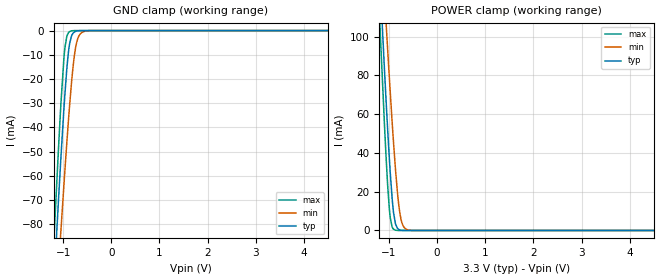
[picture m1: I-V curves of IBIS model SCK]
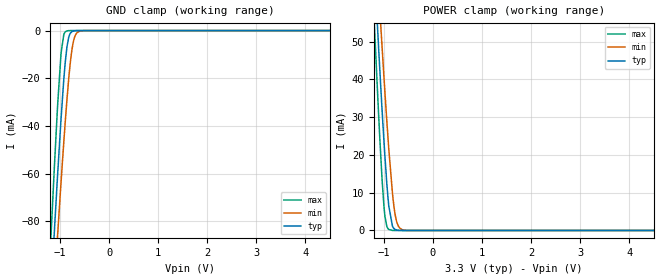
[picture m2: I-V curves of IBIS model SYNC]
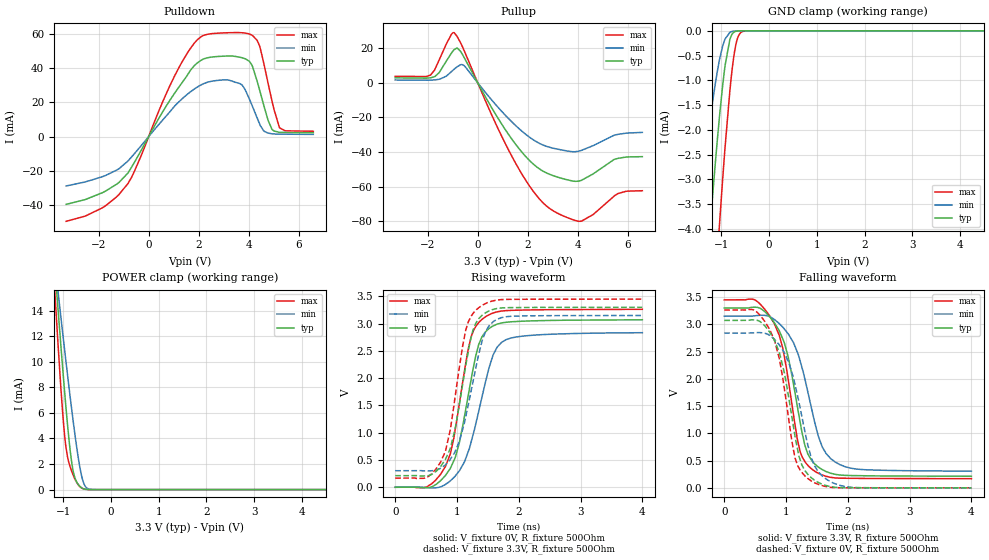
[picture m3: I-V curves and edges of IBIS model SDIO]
| Texas Instruments Incorporated
| Low-Noise Clock Jitter Cleaner with Dual Loop PLLs
| Marketing part#   Voltage Range   Package-type   #pins/pkg drawing
| LMK04826   3.0V - 3.6V   LLP   64-pin SQ
[IBIS Ver]   4.1
[File name]   lmk04826.ibs
[File Rev]   1.2
[Date]   04/24/2014
[Source]   Model built from spectre simulations at:
   Texas Instruments Incorporated.
   Analog-eLab, HPA
   12500 TI Blvd
   Dallas, TX -75243
   For Support e-mail: elab_ibis@list.ti.com
[Notes]   Revision History
   Rev 1.2: 04/24/2014
   - Correct LCPECL model name
   Rev 1.1: 01/28/2014
   - Add SYNC pin. Assign RESET to SDIO buffer
   Rev 1.0: 06/19/2013
   -Pulldown non-monotonic for LVDS_OSC model
   -Pulldown & pullup non-monotonic for LVPECL_OSC models
   -Pulldown & pullup non-monotonic for SDIO models
   -LVPECL simulation recommendation:
   It is recommended that a small (1nF or less) AC coupling cap
   be used. Larger values will result in long settling times
   - ccomp values are based on PVT settings:
   MIN: Low Voltage, High Temperature, Weak Process
   TYP: Nominal Voltage, Nominal Temperature, Nominal Process
   MAX: High Voltage, Low Temperature, Fast Process
   - C_comp although listed in numerical order of value are obtained from varying PVT conditions.
   For PVT conditions for each specific value, refer to the buffer description under respective [Model].
   IBIS model user is responsible for using appropriate C_comp to simulate for Signal Integrity.
[Disclaimer]  This model is designed as an aid for customers of Texas Instruments
 TI and its licensors and suppliers make no warranties, either expressed
 or implied, with respect to this  model, including the warranties of
 merchantability or fitness for a particular purpose.
 The model is provided solely on an "as is" basis. The entire risk as to
 its quality and performance is with the customer.
[Copyright] (C)Copyright 2014 Texas Instruments Incorporated.
   All rights reserved.
[Component]   LMK04826BISQ
[Manufacturer]  Texas Instruments Incorporated
[Package]   |64-pin LLP SQ package
|   typ   min   max
R_pkg   0   0   0
L_pkg   0   0   0
C_pkg   0   0   0
[Pin]   signal_name   model_name   R_pin   L_pin   C_pin
1   DCLKOUT0   TRI_MODE_OUT
2   DCLKOUT0*   TRI_MODE_OUT
3   SDCLKOUT1*   TRI_MODE_OUT
4   SDCLKOUT1   TRI_MODE_OUT
5   RESET   SDIO
6   SYNC   SYNC
7   NC   NC
8   NC   NC
9   NC   NC
10   VCC1   POWER
11   LDOBYP1   NC
12   LDOBYP2   NC
13   SDCLKOUT3   TRI_MODE_OUT
14   SDCLKOUT3*   TRI_MODE_OUT
15   DLKOUT2   TRI_MODE_OUT
16   DLKOUT2*   TRI_MODE_OUT
17   VCC2   POWER
18   CS   SCK
19   SCK   SCK
20   SDIO   SDIO
21   VCC3   POWER
22   SDCLKOUT5   TRI_MODE_OUT
23   SDCLKOUT5*   TRI_MODE_OUT
24   DLKOUT4   TRI_MODE_OUT
25   DLKOUT4*   TRI_MODE_OUT
26   VCC4   POWER
27   DLKOUT6   TRI_MODE_OUT
28   DLKOUT6*   TRI_MODE_OUT
29   SDCLKOUT7   TRI_MODE_OUT
30   SDCLKOUT7*   TRI_MODE_OUT
31   STATUS   SDIO
32   CPOUT1   NC
33   VCC5   POWER
34   CLKIN1   CLKIN
35   CLKIN1*   CLKIN
36   VCC6   POWER
37   CLKIN0   CLKIN
38   CLKIN0*   CLKIN
39   VCC7   POWER
40   OSCOUT   OSCOUT
41   OSCOUT*   OSCOUT
42   VCC8   POWER
43   OSCIN   OSCIN
44   OSCIN*   OSCIN
45   VCC9   POWER
46   CPOUT2   NC
47   VCC10   POWER
48   STATUS_LD2   SDIO
49   SDCLKOUT9   TRI_MODE_OUT
50   SDCLKOUT9*   TRI_MODE_OUT
51   DCLKOUT8   TRI_MODE_OUT
52   DCLKOUT8*   TRI_MODE_OUT
53   VCC11   POWER
54   DCLKOUT10   TRI_MODE_OUT
55   DCLKOUT10*   TRI_MODE_OUT
56   SDCLKOUT11   TRI_MODE_OUT
57   SDCLKOUT11*   TRI_MODE_OUT
58   CLKN_SEL0   NC
59   CLKN_SEL1   NC
60   SDCLKOUT13   TRI_MODE_OUT
61   SDCLKOUT13*   TRI_MODE_OUT
62   DCLKOUT12   TRI_MODE_OUT
63   DCLKOUT12*   TRI_MODE_OUT
64   VCC12   POWER
[Diff pin]  inv_pin  vdiff  tdelay_typ  tdelay_min  tdelay_max
 1   2   0.0   0.0s   0.0s   0.0s
 4   3   0.0   0.0s   0.0s   0.0s
13   14   0.0   0.0s   0.0s   0.0s
15   16   0.0   0.0s   0.0s   0.0s
22   23   0.0   0.0s   0.0s   0.0s
24   25   0.0   0.0s   0.0s   0.0s
27   28   0.0   0.0s   0.0s   0.0s
29   30   0.0   0.0s   0.0s   0.0s
34   35   0.0   0.0s   0.0s   0.0s
37   38   0.0   0.0s   0.0s   0.0s
40   41   0.0   0.0s   0.0s   0.0s
43   44   0.0   0.0s   0.0s   0.0s
49   50   0.0   0.0s   0.0s   0.0s
51   52   0.0   0.0s   0.0s   0.0s
54   55   0.0   0.0s   0.0s   0.0s
56   57   0.0   0.0s   0.0s   0.0s
60   61   0.0   0.0s   0.0s   0.0s
62   63   0.0   0.0s   0.0s   0.0s
[Model Selector] TRI_MODE_OUT
LVDS   LVDS OUTPUT
HSDS_6mA   HSDS 6mA OUTPUT
HSDS_8mA   HSDS 8mA OUTPUT
HSDS_10mA   HSDS 10mA OUTPUT
LVPECL1P6   LVPECL 1.6V OUTPUT
LVPECL2P0   LVPECL 2.0V OUTPUT
LCPECL   LCPECL
[Model Selector] OSCOUT
LVPECL1P6_OSC   LVPECL 1.6V OUTPUT
LVPECL2P0_OSC   LVPECL 2.0V OUTPUT
LVDS_OSC   LVDS OUTPUT
LVCMOS_OSC   LVCMOS OUTPUT
[Define Package Model]  llp64_lmk04826nsa2
[Manufacturer]  Unknown
[OEM]  Unknown
[Description]  Package Model,10GHz using buildsheet AD#LMK04826NSA2-01 RevA
[Number Of Pins]  65
[Pin Numbers]
|Pin Num   Terminal Name
1   | L1:1
2   | L2:2
3   | L3:3
4   | L4:4
5   | L5:5
6   | L6:6
7   | L7:7
8   | L8:8
9   | L9:9
10   | L10:10
11   | L11:11
12   | L12:12
13   | L13:13
14   | L14:14
15   | L15:15
16   | L16:16
17   | L17:17
18   | L18:18
19   | L19:19
20   | L20:20
21   | L21:21
22   | L22:22
23   | L23:23
24   | L24:24
25   | L25:25
26   | L26:26
27   | L27:27
28   | L28:28
29   | L29:29
30   | L30:30
31   | L31:31
32   | L32:32
33   | L33:33
34   | L34:34
35   | L35:35
36   | L36:36
37   | L37:37
38   | L38:38
39   | L39:39
40   | L40:40
41   | L41:41
42   | L42:42
43   | L43:43
44   | L44:44
45   | L45:45
46   | L46:46
47   | L47:47
48   | L48:48
49   | L49:49
50   | L50:50
51   | L51:51
52   | L52:52
53   | L53:53
54   | L54:54
55   | L55:55
56   | L56:56
57   | L57:57
58   | L58:58
59   | L59:59
60   | L60:60
61   | L61:61
62   | L62:62
63   | L63:63
64   | L64:64
65   | LDAP:65
[Model Data]
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[End Model Data]
[End Package Model]
| Models and submodels in the file (16): SCK (Input), SYNC (Input), SDIO (I/O), CLKIN (Input), OSCIN (Input), LVCMOS_OSC (Output), LVDS_OSC (Output), LVPECL1P6_OSC (Output), LVPECL2P0_OSC (Output), LVDS (Output), HSDS_6mA (Output), HSDS_8mA (Output), HSDS_10mA (Output), LVPECL1P6 (Output), LVPECL2P0 (Output), LCPECL (Output)
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|   Model SCK
[Model]   SCK
Model_type   Input
Vinl = 0.4
Vinh = 1.6
|   typ   min   max
|   (nom PVT)   (fast PVT)   (slow PVT)
C_comp   0.5966pF   0.57765pF   0.6104pF
[Voltage Range]   3.3   3.15   3.45
[Temperature Range]   27   125   -40
[Power Clamp Reference]   3.3   3.15   3.45
[GND Clamp Reference]   0   0   0
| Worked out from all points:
|   GND clamp passes 1 mA (typ) near -0.79 V on its own axis
|   POWER clamp passes 1 mA (typ) near -0.82 V on its own axis
[GND Clamp]
|   Voltage   I(typ)   I(min)   I(max)
-3.3V     -942.6mA   -854.7mA   -1.024A
-1.181V   -100.7mA   -125.5mA   -82.33mA
-1.092V   -68.4mA    -97.02mA   -46.97mA
-1.043V   -51.28mA   -81.58mA   -28.98mA
-963.6mV  -26.25mA   -57.73mA   -7.074mA
-924mV    -15.81mA   -46.4mA    -2.338mA
-864.6mV  -5.241mA   -30.59mA   -416.6uA
-785.4mV  -906.4uA   -13.39mA   -21.05uA
-726mV    -220.2uA   -5.463mA   -1.21uA
-656.7mV  -28.09uA   -1.707mA   0A
-537.9mV  -325.8nA   -217.8uA   0A
6.59V     0A         0A         0A
[POWER Clamp]
|   Voltage   I(typ)   I(min)   I(max)
-3.3V     1.303A     1.181A     1.417A
-1.191V   132mA      165.3mA    107.9mA
-1.181V   126.9mA    160.8mA    102.3mA
-1.092V   82.42mA    121.3mA    53.89mA
-1.063V   68.26mA    108.5mA    39.15mA
-993.3mV  37.62mA    79.36mA    11.46mA
-933.9mV  16.43mA    55.88mA    1.777mA
-864.6mV  3.384mA    31.47mA    134.7uA
-805.2mV  682.9uA    15.13mA    8.179uA
-745.8mV  107.4uA    5.402mA    0A
-577.5mV  0A         144uA      0A
6.59V     0A         0A         0A
|   Model   SYNC
[Model]   SYNC
Model_type   Input
Vinl = 0.4
Vinh = 1.2
|   typ   min   max
|   (nom PVT)   (fast PVT)   (slow PVT)
C_comp   0.1841pF   0.1807pF   0.1863pF
[Voltage Range]   3.3   3.15   3.45
[Temperature Range]   27   125   -40
[Power Clamp Reference]   3.3   3.15   3.45
[GND Clamp Reference]   0   0   0
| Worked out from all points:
|   GND clamp passes 1 mA (typ) near -0.79 V on its own axis
|   POWER clamp passes 1 mA (typ) near -0.82 V on its own axis
[GND Clamp]
|   Voltage   I(typ)   I(min)   I(max)
-3.3V     -965.6mA   -893.6mA   -1.069A
-1.191V   -112.1mA   -132.7mA   -88.59mA
-1.117V   -84.4mA    -107.7mA   -57.4mA
-1.048V   -59.55mA   -84.92mA   -30.5mA
-978.5mV  -36.37mA   -62.95mA   -9.221mA
-924mV    -20.4mA    -46.56mA   -1.598mA
-859.7mV  -6.75mA    -28.81mA   -125.9uA
-795.3mV  -1.278mA   -14.16mA   -6.167uA
-735.9mV  -231.4uA   -5.307mA   -320.6nA
-681.5mV  -39.54uA   -1.674mA   -17.85nA
-577.5mV  -941.8nA   -148.2uA   0A
6.595V    0A         0A         0A
[POWER Clamp]
|   Voltage   I(typ)   I(min)   I(max)
-3.3V     638.8mA    590.5mA    708.3mA
-1.196V   70.39mA    83.75mA    55.37mA
-1.107V   48.47mA    63.9mA     30.8mA
-1.077V   41.42mA    57.43mA    23.19mA
-1.038V   32.31mA    48.95mA    13.93mA
-978.5mV  19.65mA    36.67mA    3.829mA
-899.2mV  6.493mA    21.57mA    264.8uA
-825mV    1.174mA    9.968mA    10.77uA
-765.6mV  254.2uA    3.922mA    572nA
-701.3mV  35.15uA    1.11mA     20.08nA
-582.5mV  493.7nA    81.77uA    0A
6.595V    0A         0A         0A
|   Model SDIO
[Model]   SDIO
Model_type   I/O
Polarity   Non-Inverting
Enable   Active-Low
Vinl = 0.4
Vinh = 1.6
Vmeas = 1.65
Vref = 3.3
Cref = 15pF
Rref = 500
|   typ   min   max
|   (nom PVT)   (Fast PVT)   (slow PVT)
C_comp   0.555p   0.552p   0.559p
|C_comp (ON state)   0.555p   0.552p   0.559p
|C_comp (OFF state)   0.540p   0.535p   0.544p
| Where   nom PVT is  Nominal Process, 3.3V, 27C
|   Fast PVT is Strong Process, 3.45V, -40C
|   Slow PVT is Weak Process, 3.15V, 125C
[Voltage Range]   3.3   3.15   3.45
[Temperature Range]   27   125   -40
[Pullup Reference]   3.3   3.15   3.45
[Pulldown Reference]   0   0   0
[Power Clamp Reference]   3.3   3.15   3.45
[GND Clamp Reference]   0   0   0
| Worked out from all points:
|   slope of the pulldown table from 0 to 0.495 V, typ, clamps not added: 38.6 ohm
|   slope of the pullup table from 0 to 0.495 V, typ, clamps not added: 38.7 ohm
|   GND clamp passes 1 mA (typ) near -0.96 V on its own axis
|   POWER clamp passes 1 mA (typ) near -0.76 V on its own axis
|   falling waveform, V_fixture 3.3V, R_fixture 500Ohm: 20-80 % time 329ps typ, 396ps min, 304ps max; typ from 3.3 V to 0.213 V
|   rising waveform, V_fixture 0V, R_fixture 500Ohm: 20-80 % time 326ps typ, 386ps min, 298ps max; typ from 0 V to 3.07 V
|   rising waveform, V_fixture 3.3V, R_fixture 500Ohm: 20-80 % time 298ps typ, 337ps min, 281ps max; typ from 0.213 V to 3.3 V
|   falling waveform, V_fixture 0V, R_fixture 500Ohm: 20-80 % time 306ps typ, 352ps min, 293ps max; typ from 3.07 V to 0 V
[Pulldown]
|   Voltage   I(typ)   I(min)   I(max)
-3.3V     -39.51mA   -28.78mA   -49.4mA
-1.855V   -32.74mA   -23.4mA    -41.56mA
-825mV    -21.19mA   -14.19mA   -27.32mA
1.115V    26.94mA    18.95mA    37.59mA
1.808V    41.12mA    27.59mA    54.16mA
2.224V    45.44mA    31.04mA    59.18mA
3.67V     46.25mA    30.83mA    60.66mA
4.165V    40.64mA    17.32mA    58.9mA
4.442V    27.14mA    7.375mA    52.86mA
4.778V    9.588mA    2.062mA    31.25mA
5.234V    2.507mA    1.461mA    5.294mA
6.59V     2.258mA    1.308mA    3.132mA
[GND Clamp]
|   Voltage   I(typ)   I(min)   I(max)
-3.3V     -32.55mA   -22.55mA   -41.85mA
-1.498V   -7.359mA   -3.9mA     -11.04mA
-1.261V   -4.258mA   -1.969mA   -7.206mA
-1.181V   -3.287mA   -1.408mA   -5.977mA
-1.043V   -1.747mA   -592.8uA   -3.933mA
-924mV    -700.9uA   -165.3uA   -2.348mA
-795.3mV  -102.4uA   -18.88uA   -946.5uA
-735.9mV  -26.69uA   -5.763uA   -488.3uA
-676.5mV  -5.707uA   -1.635uA   -195.9uA
-617.1mV  -1.054uA   -434.4nA   -59.58uA
-518.1mV  0A         0A         -5.761uA
6.59V     0A         0A         0A
[Pullup]
|   Voltage   I(typ)   I(min)   I(max)
-3.3V     2.838mA    1.604mA    3.746mA
-1.884V   2.87mA     1.509mA    4.457mA
-1.548V   5.78mA     2.005mA    12.97mA
-943.8mV  19.07mA    7.823mA    28.97mA
-825mV    20.11mA    9.247mA    26.79mA
-537.9mV  14.47mA    9.821mA    18.44mA
1.393V    -33.02mA   -22.93mA   -43.08mA
2.175V    -46.23mA   -32.41mA   -61.62mA
2.779V    -52.18mA   -36.79mA   -71.39mA
4.135V    -56.37mA   -39.1mA    -79.87mA
5.61V     -43.62mA   -29.77mA   -63.95mA
6.59V     -42.62mA   -28.62mA   -62.29mA
[POWER Clamp]
|   Voltage   I(typ)   I(min)   I(max)
-3.3V     125mA      90.16mA    153.8mA
-1.181V   17.55mA    17.82mA    15.64mA
-1.171V   17.06mA    17.48mA    15.02mA
-1.132V   15.11mA    16.15mA    12.59mA
-1.082V   12.71mA    14.5mA     9.663mA
-1.003V   8.987mA    11.89mA    5.49mA
-943.8mV  6.36mA     9.97mA     3.265mA
-854.7mV  2.98mA     7.172mA    1.743mA
-795.3mV  1.474mA    5.393mA    1.144mA
-587.4mV  82.22uA    656.7uA    72.92uA
-399.3mV  793.6nA    8.386uA    949.6nA
6.59V     0A         0A         0A
[Ramp]
R_load = 500
|   typ   min   max
dV/dt_r   1.84196/3.25658e-10   1.70003/3.86019e-10   1.95703/2.97502e-10
dV/dt_f   1.85143/3.29443e-10   1.70554/3.95766e-10   1.96811/3.03724e-10
[Falling Waveform]
V_fixture = 3.3V
V_fixture_min = 3.15V
V_fixture_max = 3.45V
R_fixture = 500Ohm
C_fixture = 0F
|   Time   V(typ)   V(min)   V(max)
0s        3.299V     3.149V     3.449V
481.2ps   3.314V     3.155V     3.455V
812ps     3.028V     3.089V     3.009V
948.1ps   2.728V     2.946V     2.557V
1.034ns   2.406V     2.826V     1.994V
1.228ns   1.204V     2.327V     664.1mV
1.407ns   517.3mV    1.486V     353.4mV
1.585ns   336.4mV    753.8mV    236.8mV
1.87ns    237mV      427.5mV    178mV
4ns       213.5mV    306.8mV    168.7mV
[Rising Waveform]
V_fixture = 0V
V_fixture_min = 0V
V_fixture_max = 0V
R_fixture = 500Ohm
C_fixture = 0F
|   Time   V(typ)   V(min)   V(max)
0s        216.6uV    221.7uV    222.7uV
509.6ps   -8.212mV   -6.487mV   6.985mV
732ps     117.5mV    8.278mV    234.2mV
891.1ps   344.8mV    117.6mV    610.2mV
1.034ns   799.5mV    296.5mV    1.506V
1.228ns   1.975V     828.2mV    2.758V
1.407ns   2.762V     1.669V     3.08V
1.585ns   2.957V     2.427V     3.194V
1.794ns   3.024V     2.706V     3.238V
4ns       3.07V      2.834V     3.262V
[Rising Waveform]
V_fixture = 3.3V
V_fixture_min = 3.15V
V_fixture_max = 3.45V
R_fixture = 500Ohm
C_fixture = 0F
|   Time   V(typ)   V(min)   V(max)
0s        212.6mV    303.6mV    168.4mV
509.6ps   210.1mV    298.2mV    181.1mV
811.1ps   506.7mV    410mV      653.1mV
971.1ps   1.077V     660.1mV    1.669V
1.145ns   2.25V      1.312V     2.895V
1.256ns   2.87V      1.917V     3.18V
1.354ns   3.093V     2.448V     3.294V
1.522ns   3.233V     2.964V     3.395V
1.723ns   3.287V     3.111V     3.44V
4ns       3.299V     3.149V     3.449V
[Falling Waveform]
|Gnd
V_fixture = 0V
V_fixture_min = 0V
V_fixture_max = 0V
R_fixture = 500Ohm
C_fixture = 0F
|   Time   V(typ)   V(min)   V(max)
0s        3.072V     2.84V      3.263V
509.6ps   3.078V     2.846V     3.243V
811.1ps   2.711V     2.727V     2.711V
971.1ps   2.12V      2.478V     1.831V
1.145ns   950.5mV    1.899V     551.8mV
1.256ns   420.8mV    1.309V     284.7mV
1.354ns   247.1mV    779.5mV    170.5mV
1.522ns   99.93mV    295.9mV    65.69mV
1.87ns    5.268mV    46.54mV    2.417mV
4ns       321.9uV    459.9uV    306.4uV
